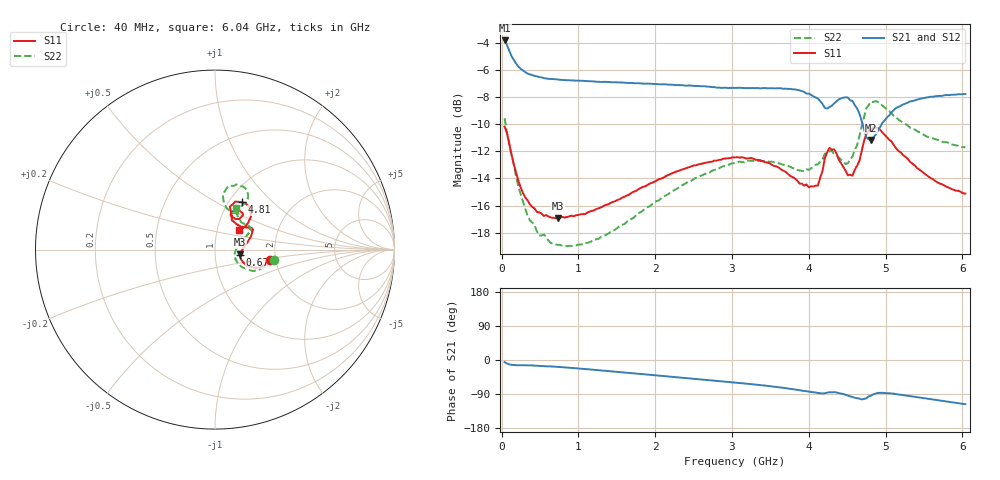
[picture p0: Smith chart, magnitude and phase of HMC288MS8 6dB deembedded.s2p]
!Hittite Microwave Corporation
!12 Elizabeth Drive
!Chelmsford, MA 01824
!Tel: 978-250-3343
!Fax: 978-250-3373
!Device: HMC288MS8, 0.7-3.7 GHz GaAs IC 3-bit Digital Attenuator in 8-lead Grounded Base surface Mount Plastic Package
!Misc:  6dB state, room
# GHZ S DB R 50.0
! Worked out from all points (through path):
!   201 points, 40 MHz to 6.04 GHz, reference 50 ohm
!   highest |S21| = -3.84 dB at 40 MHz (marker M1); lowest = -11.2 dB at 4.81 GHz (marker M2)
!   group delay of S21, straight-line fit = 49.7 ps
!   lowest |S11| = -16.9 dB at 730 MHz (marker M3), VSWR 1.33, Z = 66.1 - j3.66 ohm
!   |S11| at or under -10 dB: start of sweep to end of sweep
!   |S22| runs from -19.0 to -8.3 dB; largest |S21 - S12| = 0.0039
!   S11 on the Smith chart (normalised r, x): 40 MHz: 1.85, -0.24; 670 MHz: 1.32, -0.08; 4.81 GHz: 1.14, +0.67; 6.04 GHz: 1.28, +0.29
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0.04  -10.19 -10.8  -3.84 -5.6  -3.83 -5.4  -9.57 -10.5
0.13  -12.24 -24.5  -5.00 -12.8  -4.95 -12.5  -12.28 -29.4
0.34  -15.62 -22.9  -6.29 -14.1  -6.27 -14.1  -16.75 -30.1
0.49  -16.50 -17.9  -6.54 -15.6  -6.51 -15.6  -18.20 -25.7
0.67  -16.90 -12.3  -6.68 -17.4  -6.69 -17.4  -18.80 -17.9
0.73  -16.95 -11.0  -6.71 -18.1  -6.72 -18.2  -18.90 -15.3
1.06  -16.63 -3.0  -6.81 -23.4  -6.81 -23.4  -18.84 -3.9
2.05  -14.06 16.6  -7.06 -41.2  -7.05 -41.3  -15.61 19.3
3.04  -12.45 28.8  -7.34 -59.4  -7.31 -59.6  -12.89 29.5
3.58  -13.12 33.7  -7.37 -71.2  -7.35 -71.3  -12.82 35.6
4.06  -14.60 53.9  -7.96 -85.3  -7.94 -85.4  -13.15 53.8
4.12  -14.53 60.0  -8.11 -87.1  -8.09 -87.3  -12.98 56.0
4.18  -13.45 65.9  -8.52 -88.7  -8.49 -88.9  -12.59 58.7
4.27  -11.76 58.2  -8.74 -85.0  -8.74 -85.2  -12.01 56.9
4.36  -12.13 51.0  -8.33 -85.7  -8.29 -85.7  -12.30 56.9
4.51  -13.77 56.0  -8.05 -94.1  -8.06 -94.2  -12.88 67.9
4.57  -13.81 60.7  -8.29 -97.5  -8.32 -97.7  -12.39 74.3
4.69  -11.97 71.0  -9.78 -104.2  -9.74 -104.7  -10.15 81.9
4.81  -10.36 60.6  -11.16 -94.3  -11.22 -94.8  -8.36 72.1
5.05  -11.16 44.3  -9.34 -87.8  -9.29 -87.8  -9.05 58.5
5.47  -13.47 37.8  -8.11 -99.9  -8.10 -100.0  -10.70 58.4
6.04  -15.12 39.4  -7.78 -116.7  -7.77 -116.8  -11.71 63.6
